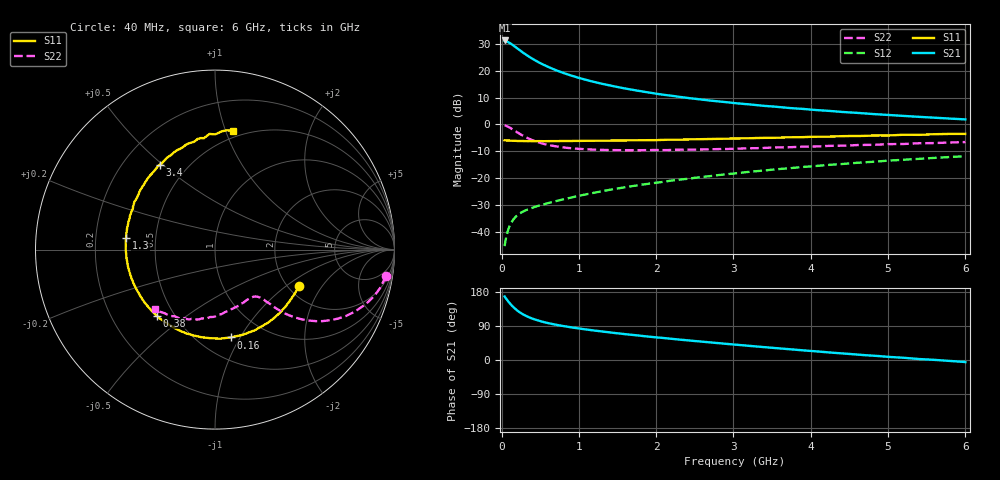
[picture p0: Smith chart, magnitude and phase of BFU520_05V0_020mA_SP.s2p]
! Filename:  P:\Prog\Test\Noise\ATS_data\Testdata_Net\03 Spar\BFU520_APG2013_37_A05_05p0V_020mA_SP_CM01_D.s2p
! Date/Time: Fri 26/Apr/2013 13:00:09
! BFU520_APG2013_37_A05_05p0V_1to20mA_SP_CM01_Bias8_R.s2p
! MDIF S-parameter v. bias file
! BFU520_APG2013_37_A05_05p0V_1to20mA_SP_CM01
! Date/time Tue Apr 23 15:26:19 2013
! VAR V_out= 5.0010
! VAR I_out= 20.0000
! VAR V_in= 0.8453
! VAR I_in= 0.2344
! Device data file deembeded for feedlines and parallel
! Original file: \03 Spar\BFU520_APG2013_37_A05_05p0V_020mA_SP_CM01_R.s2p
! Feed-files: PR047V01_250413_Feed1.s2p, PR047V01_250413_Feed2.s2p
! Parallel-file: PR047V01_250413_Par.s2p
# MHz S MA R 50
!  Freq-MHz  S11-mag  S11-arg  S21-mag  S21-arg  S12-mag  S12-arg  S22-mag  S22-arg
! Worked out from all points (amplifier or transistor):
!   98 points, 40 MHz to 6 GHz, reference 50 ohm
!   highest |S21| = 31.2 dB at 40 MHz (marker M1)
!   |S21| within 3 dB of that: start of sweep to 206.2 MHz
!   unconditionally stable (mu >= 1): 1.229 GHz to 3.19 GHz
!   at 300 MHz: K = 0.48, MSG = 29.2 dB, |S12| = -32.1 dB
!   at 1.6 GHz: K = 1.05, MAG = 17.0 dB, |S12| = -23.3 dB
!   at 6 GHz: K = 0.81, MSG = 6.8 dB, |S12| = -11.8 dB
!   S11 on the Smith chart (normalised r, x): 40 MHz: 2.30, -1.24; 160 MHz: 0.70, -0.91; 380 MHz: 0.40, -0.39; 1.3 GHz: 0.34, +0.06; 3.4 GHz: 0.35, +0.49; 6 GHz: 0.44, +1.06
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40  0.5095 -23.1  36.5 167.7  0.005471 82.1  0.9634 -8.8
50  0.5075 -28.8  36.32 164.2  0.006713 79.7  0.9541 -10.9
90  0.5037 -49.6  33.76 153.8  0.01142 72.4  0.9015 -18.9
120  0.5011 -63.7  31.84 146.6  0.01437 67.8  0.8517 -24.0
140  0.4991 -72.1  30.41 142.2  0.01608 65.2  0.8179 -26.9
160  0.4971 -79.8  28.91 138.2  0.01764 63.0  0.7847 -29.4
200  0.4944 -93.2  26.21 131.2  0.02023 59.5  0.7201 -33.6
260  0.4934 -109.4  22.68 122.7  0.02326 56.2  0.6393 -37.9
320  0.4913 -121.7  19.75 116.0  0.02566 54.4  0.5753 -40.7
380  0.491 -131.4  17.35 110.8  0.02768 53.6  0.525 -42.5
480  0.4907 -143.6  14.36 103.9  0.03088 53.6  0.4649 -44.0
600  0.4904 -154.5  11.84 97.5  0.03447 54.7  0.4187 -45.0
800  0.4932 -167.1  9.09 89.6  0.04065 56.9  0.3751 -46.4
1050  0.4966 -178.8  7.029 81.8  0.04882 59.1  0.3493 -48.6
1300  0.4996 172.4  5.719 75.2  0.05744 60.6  0.3373 -51.5
1600  0.5051 163.1  4.665 68.2  0.06813 61.4  0.3327 -55.9
2050  0.5157 152.4  3.648 58.9  0.08431 61.6  0.3344 -63.6
3100  0.5512 129.1  2.435 39.2  0.1269 58.6  0.3575 -82.7
3400  0.5645 122.9  2.218 33.9  0.1396 56.9  0.3668 -88.4
4100  0.5932 110.5  1.843 22.3  0.1708 52.5  0.3915 -101.2
5200  0.6453 92.7  1.444 5.9  0.2212 44.1  0.4342 -121.2
6000  0.6686 81.4  1.244 -5.3  0.2574 36.8  0.4719 -135.3
